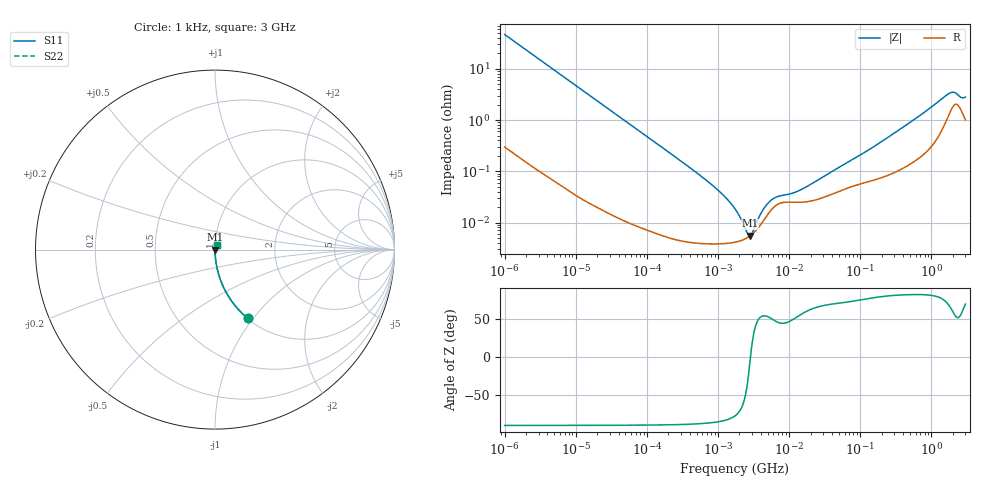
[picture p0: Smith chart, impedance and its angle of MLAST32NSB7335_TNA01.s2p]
! MLAST32NSB7335_TNA01  S-PARAMETER MODEL  ( Standard Model )
! Model Generated by TAIYO YUDEN Corporation (http://www.ty-top.com)
! Version 1.0
! TAIYO YUDEN Control No. 220601
! Copyright(c) 2009 TAIYO YUDEN CO.,LTD. All Rights Reserved.
! Product Description (link to TY-COMPAS)
! https://ds.yuden.co.jp/TYCOMPAS/or/detail?pn=MLAST32NSB7335KTNA01&u=M
! Products Name : Multilayer Ceramic Capacitors
! Characteristics :
!  Capacitance : 3.3 [uF] , Rated Voltage : 25 [V] , TCC : X7R
!  Case Size : 3.2 x 2.5 / 0.126 x 0.098 [mm/inch] , Thickness : 1.9 / 0.075 [mm/inch]
!  (Conditions: Temperature = 25 [degC] , DC Bias Voltage = 0 [V])
! External Node Assignments :
!  1  o---| |---o  2
! GND o---------o GND
! Frequency Range : 1kHz  -  3GHz  [ 401 STEP ]
# MHZ S RI R 50
! Freq[MHz].  S11 Real  S11 Imag  S21 Real  S21 Imag  S12 Real  S12 Imag  S22 Real  S22 Imag
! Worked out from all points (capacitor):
!   401 points, 1 kHz to 3 GHz, reference 50 ohm
!   read as one part in series: C = 3.38 uF near 1.077 kHz
!   lowest |Z| = 5.5 mohm at 2.812 MHz (marker M1)
!   series resonance near 2.862 MHz, so ESL is about 910 pH
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0.001  0.1824 -0.383  0.8176 0.383  0.8176 0.383  0.1824 -0.383
0.001564  0.0845 -0.275  0.9155 0.275  0.9155 0.275  0.0845 -0.275
0.002447  0.0369 -0.1854  0.9631 0.1854  0.9631 0.1854  0.0369 -0.1854
0.004969  0.0096 -0.0942  0.9904 0.0942  0.9904 0.0942  0.0096 -0.0942
0.01216  0.00181 -0.039  0.9982 0.039  0.9982 0.039  0.00181 -0.039
0.147855  6.88e-05 -0.00324  0.9999 0.00324  0.9999 0.00324  6.88e-05 -0.00324
0.821683  3.85e-05 -0.000542  1 0.000542  1 0.000542  3.85e-05 -0.000542
1.285341  3.91e-05 -0.000304  1 0.000304  1 0.000304  3.91e-05 -0.000304
1.732051  4.12e-05 -0.000181  1 0.000181  1 0.000181  4.12e-05 -0.000181
2.24859  4.59e-05 -8.49e-05  1 8.49e-05  1 8.49e-05  4.59e-05 -8.49e-05
2.812335  5.47e-05 -6.07e-06  0.9999 6.07e-06  0.9999 6.07e-06  5.47e-05 -6.07e-06
3.264662  6.55e-05 4.68e-05  0.9999 -4.68e-05  0.9999 -4.68e-05  6.55e-05 4.68e-05
3.517417  7.34e-05 7.33e-05  0.9999 -7.33e-05  0.9999 -7.33e-05  7.34e-05 7.33e-05
4.566395  0.00012 0.000162  0.9999 -0.000162  0.9999 -0.000162  0.00012 0.000162
5.928204  0.000192 0.000218  0.9998 -0.000218  0.9998 -0.000218  0.000192 0.000218
12.49624  0.000248 0.000309  0.9998 -0.000309  0.9998 -0.000309  0.000248 0.000309
21.06097  0.000266 0.000514  0.9997 -0.000514  0.9997 -0.000514  0.000266 0.000514
256.0921  0.000878 0.00471  0.9991 -0.00471  0.9991 -0.00471  0.000878 0.00471
1780.008  0.0139 0.0298  0.9861 -0.0298  0.9861 -0.0298  0.0139 0.0298
2066.299  0.0198 0.028  0.9802 -0.028  0.9802 -0.028  0.0198 0.028
2584.342  0.0163 0.0221  0.9837 -0.0221  0.9837 -0.0221  0.0163 0.0221
3000  0.0107 0.0258  0.9893 -0.0258  0.9893 -0.0258  0.0107 0.0258
